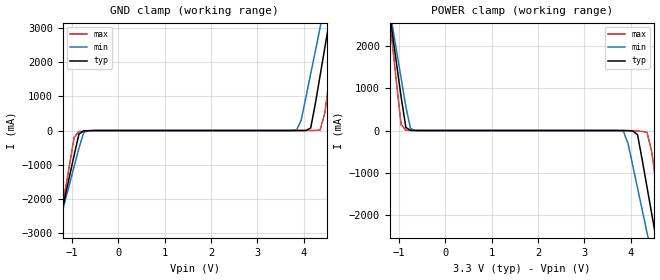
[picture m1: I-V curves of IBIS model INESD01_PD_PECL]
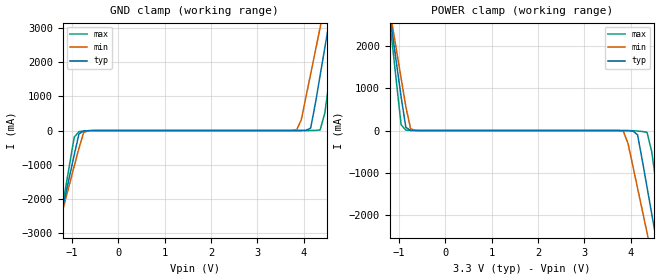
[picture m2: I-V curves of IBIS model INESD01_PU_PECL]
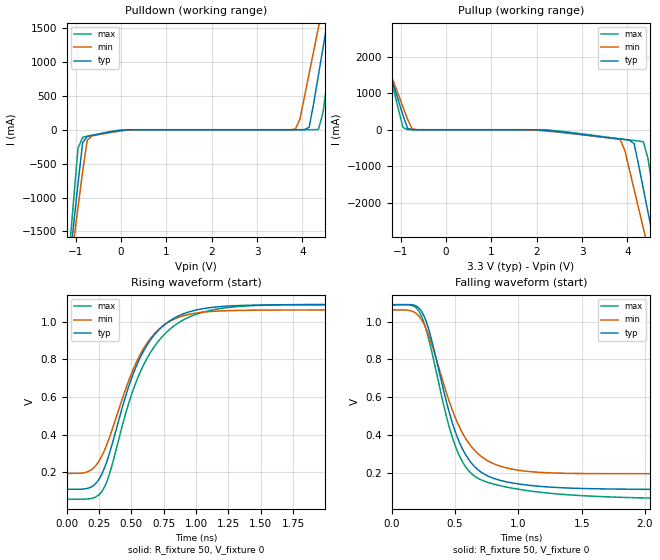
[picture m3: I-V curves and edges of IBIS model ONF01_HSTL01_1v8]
|   This file is an IBIS representation of the   |
|   Integrated Device Technology , Inc.   |
|   ICS8725-21   |
|   DIFFERENTIAL-TO-HSTL ZERO DELAY CLOCK GENERATOR   |
[IBIS Ver]   4.1
[File name]   8725_21_3v3.ibs
[File Rev]   2.0
[Date]   2 Sep 2009 | Last modified
|   2 Jul 2002 | Generated
[Source]   Originated at Integrated Device Technology, Inc.
[Disclaimer]
IDT hereby grants the user of this IBIS model a non-exclusive,
nontransferable license to use this IBIS model under the following terms.
Before using this IBIS model, the user should read this license.
If the user does not accept these terms,  the IBIS model should be
returned to IDT within 30 days.
   The user is granted this license only to use the IBIS model and
is not granted rights to sell, load, rent, lease or license the IBIS
model in whole or in part, or in modified form to anyone other than
user. User may modify the IBIS model to suit its specific
applications but rights to derivative works and such modifications
shall belong to IDT.
   This IBIS model is provided on an "AS IS" basis and IDT makes
absolutely no warranty with respect to the information contained
herein. IDT DISCLAIMS AND CUSTOMER WAIVES ALL WARRANTIES, EXPRESS
OR IMPLIED, INCLUDING WARRANTIES OF MERCHANTABILITY OR FITNESS FOR
A PARTICULAR PURPOSE. The entire risk as to quality and performance
is with the Customer. ACCORDINGLY, IN NO EVENT SHALL THE COMPANY BE
LIABLE FOR ANY DAMAGES, WHETHER IN CONTRACT OR TORT,INCLUDING ANY
LOST PROFITS OR OTHER INCIDENTAL, CONSEQUENTIAL, EXEMPLARY, OR
PUNITIVE DAMAGES ARISING OUT OF THE USE OR APPLICATION OF THE IBIS
model provided in this package. Further, IDT reserves the right to
make changes without notice to any product herein to improve
reliability, function, or design. IDT does not convey any license
under patent rights or any other intellectual property rights,
including those of third parties.
   IDT is not obligated to provide maintenance or support
for the licensed IBIS model.
[Copyright]   Copyright 2002 by Integrated Device Technology , Inc.
[Component]   8725M_21
[Manufacturer] Integrated Device Technology, Inc.
[Package]
|SOIC 20 Lead
|   typ   min   max
R_pkg   57.15m   45.4m   68.9m
L_pkg   4.051n   2.187n   5.914n
C_pkg   0.796p   0.419p   1.173p
[Pin]  signal_name   model_name   R_pin   L_pin   C_pin
1   CLK   INESD01_PD_PECL   68.90m   5.914n   1.173p
2   nCLK   INESD01_PU_PECL   63.02m   4.983n   0.985p
3   MR   INESD01_PD_PECL   57.15m   4.051n   0.796p
4   VDD   POWER   51.25m   3.119n   0.608p
5   nFB_IN   INESD01_PU_PECL   45.40m   2.187n   0.419p
6   FB_IN   INESD01_PD_PECL   45.40m   2.187n   0.419p
7   SEL2   INESD01_PD_PECL   51.25m   3.119n   0.608p
8   GND   GND   57.15m   4.051n   0.796p
9   nQFB   ONF01_HSTL01_1v8   63.02m   4.983n   0.985p
10   QFB   ONF01_HSTL01_1v8   68.90m   5.914n   1.173p
11   nQ   ONF01_HSTL01_1v8   68.90m   5.914n   1.173p
12   Q   ONF01_HSTL01_1v8   63.02m   4.983n   0.985p
13   VDDO   POWER   57.15m   4.051n   0.796p
14   SEL3   INESD01_PD_PECL   51.25m   3.119n   0.608p
15   VDDA   POWER   45.40m   2.187n   0.419p
16   PLL_SEL   INESD01_PU_PECL   45.40m   2.187n   0.419p
17   VDD   POWER   51.25m   3.119n   0.608p
18   SEL0   INESD01_PD_PECL   57.15m   4.051n   0.796p
19   SEL1   INESD01_PD_PECL   63.02m   4.983n   0.985p
20   NC   NC   68.90m   5.914n   1.173p
[Diff Pin]  inv_pin  vdiff tdelay_typ tdelay_min  tdelay_max
|Output
10   9   NA   0   0   0
12   11   NA   0   0   0
|Input
1   2   0.15   0   0   0
6   5   0.15   0   0   0
| Models and submodels in the file (3): INESD01_PD_PECL (Input), INESD01_PU_PECL (Input), ONF01_HSTL01_1v8 (Output)
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[Model]   INESD01_PD_PECL
Model_type  Input
Polarity   Non-Inverting
Vinl = 0.8V
Vinh = 2.0V
|   typ   min   max
C_comp   2pF   1.5pF   2.5pF
|   typ   min   max
[Voltage range]  3.3V   3.15V   3.45V
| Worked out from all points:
|   GND clamp passes 1 mA (typ) near -0.55 V on its own axis
|   POWER clamp passes 1 mA (typ) near -0.66 V on its own axis
[GND_clamp]
|Voltage   I(typ)   I(min)   I(max)
-2.586V   -10.86A    -9.487A    -13.15A
-1.361V   -3.24A     -3.145A    -3.432A
-1.259V   -2.606A    -2.617A    -2.622A
-952.6mV  -705.3mA   -1.038A    -192.4mA
-850.5mV  -99.9mA    -513.5mA   -31.23mA
-646.4mV  -3.788mA   -3.549mA   -8.297mA
3.844V    129.1uA    13.13mA    71.12uA
4.151V    73.33mA    1.652A     864.7uA
4.355V    1.607A     3.003A     15.44mA
4.559V    3.233A     4.356A     1.553A
4.763V    4.861A     5.711A     3.635A
5.375V    9.757A     9.783A     9.893A
[POWER_clamp]
|Voltage   I(typ)   I(min)   I(max)
-2.177V   10.57A     9.364A     12.62A
-1.157V   2.42A      2.586A     2.194A
-952.6mV  795.8mA    1.237A     137.8mA
-850.5mV  73.33mA    563.2mA    8.145mA
-646.4mV  535.8uA    2.004mA    431.2uA
3.844V    -826.3uA   -18.14mA   -47.07uA
4.151V    -99.9mA    -1.362A    -11.82mA
4.355V    -1.338A    -2.415A    -41.71mA
4.559V    -2.606A    -3.47A     -1.312A
4.661V    -3.24A     -3.998A    -2.123A
4.763V    -3.875A    -4.526A    -2.933A
5.579V    -8.954A    -8.756A    -9.414A
[Model]   INESD01_PU_PECL
Model_type  Input
Polarity   Non-Inverting
Vinl = 0.8V
Vinh = 2.0V
|   typ   min   max
C_comp   2pF   1.5pF   2.5pF
|   typ   min   max
[Voltage range]  3.3V   3.15V   3.45V
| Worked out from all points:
|   GND clamp passes 1 mA (typ) near -0.55 V on its own axis
|   POWER clamp passes 1 mA (typ) near -0.67 V on its own axis
[GND_clamp]
|Voltage   I(typ)   I(min)   I(max)
-3.3V     -15.3A     -13.19A    -18.82A
-1.361V   -3.24A     -3.145A    -3.432A
-1.259V   -2.606A    -2.617A    -2.622A
-952.6mV  -705.4mA   -1.038A    -192.5mA
-850.5mV  -99.96mA   -513.6mA   -31.29mA
-646.4mV  -3.852mA   -3.611mA   -8.361mA
3.844V    64.83uA    13.07mA    7.183uA
4.151V    73.26mA    1.652A     800.8uA
4.355V    1.607A     3.003A     15.37mA
4.559V    3.233A     4.356A     1.553A
4.763V    4.861A     5.711A     3.635A
6.6V      19.56A     17.94A     22.42A
[POWER_clamp]
|Voltage   I(typ)   I(min)   I(max)
-3.3V     19.56A     16.84A     24.11A
-1.259V   3.233A     3.262A     3.235A
-1.157V   2.419A     2.586A     2.194A
-952.6mV  795.8mA    1.236A     137.7mA
-850.5mV  73.26mA    563.1mA    8.081mA
-646.4mV  471.5uA    1.942mA    367.2uA
3.844V    -890.5uA   -18.21mA   -111uA
4.151V    -99.96mA   -1.362A    -11.88mA
4.355V    -1.338A    -2.415A    -41.77mA
4.559V    -2.606A    -3.47A     -1.313A
4.763V    -3.875A    -4.526A    -2.933A
6.6V      -15.3A     -14.05A    -17.51A
[Model]   ONF01_HSTL01_1v8
|3.3V core, 1.8V output supply
Model_type  Output
Polarity   Non-Inverting
Vmeas = .6
Rref = 50
Cref = 0
Vref = 0
|Variable  typ   min   max
C_comp   2p   1.5p   2.5p
[Voltage Range]   3.3   3.135   3.465
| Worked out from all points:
|   slope of the pulldown table from 0 to 0.495 V, typ, clamps not added: 54.9 ohm
|   rising waveform, R_fixture 50, V_fixture 0: 20-80 % time 306ps typ, 302ps min, 333ps max; typ from 0.111 V to 1.09 V
|   falling waveform, R_fixture 50, V_fixture 0: 20-80 % time 255ps typ, 284ps min, 252ps max; typ from 1.09 V to 0.111 V
| Open source, no load
|  Voltage   I(typ)   I(min)   I(max)
[Pulldown]
-3.3V     -15.42A    -13.35A    -18.91A
-1.157V   -2.072A    -2.21A     -1.894A
-1.055V   -1.436A    -1.68A     -1.084A
-952.6mV  -800.4mA   -1.149A    -274.1mA
-850.5mV  -191.4mA   -618.4mA   -111.9mA
-544.3mV  -70.23mA   -78.22mA   -68.72mA
3.844V    27.09uA    7.698mA    3.013nA
4.151V    36.63mA    830.7mA    49.54uA
4.355V    803.8mA    1.508A     4.53mA
4.559V    1.617A     2.187A     770.5mA
4.763V    2.432A     2.867A     1.809A
6.6V      9.786A     9.002A     11.19A
[Pullup]
-3.3V     9.786A     8.45A      12.03A
-1.565V   2.839A     2.657A     3.17A
-1.463V   2.432A     2.317A     2.65A
-952.6mV  398mA      622.1mA    64.71mA
-850.5mV  36.63mA    284.2mA    1.532mA
-646.4mV  229.4uA    1.613mA    19.07uA
3.844V    -256mA     -270.5mA   -249.6mA
4.151V    -379.9mA   -1.636A    -294.5mA
4.355V    -1.626A    -2.699A    -329.8mA
4.559V    -2.898A    -3.761A    -1.602A
4.763V    -4.17A     -4.823A    -3.222A
6.6V      -15.62A    -14.38A    -17.8A
[Ramp]
|   typ   min   max
dV/dt_r   0.782/0.488n   0.693/0.472n   0.826/0.535n
dV/dt_f   0.783/0.418n   0.693/0.453n   0.822/0.447n
R_load =   50.0000
[Rising Waveform]
R_fixture = 50
V_fixture = 0
C_fixture = 0.0p
| Time   typ   min   max
0s        110.9mV    195.1mV    57.72mV
173.6ps   118.9mV    207.8mV    60.43mV
275.9ps   199mV      294.5mV    104.4mV
334.8ps   312.4mV    395.2mV    202.7mV
480.5ps   659.8mV    690.1mV    570.6mV
579.7ps   826mV      840.3mV    750.2mV
728.5ps   967.2mV    969.3mV    912.9mV
917.6ps   1.045V     1.034V     1.015V
1.423ns   1.087V     1.06V      1.084V
2.998ns   1.089V     1.062V     1.089V
[Falling Waveform]
R_fixture = 50
V_fixture = 0
C_fixture = 0.0p
| Time   typ   min   max
0s        1.089V     1.062V     1.088V
170.5ps   1.087V     1.052V     1.083V
244.9ps   1.042V     999.2mV    1.011V
303.8ps   931.1mV    904.4mV    875.3mV
421.6ps   601.8mV    644.6mV    525.1mV
492.9ps   434.4mV    506.4mV    359mV
582.8ps   296.3mV    382.4mV    232.4mV
691.3ps   210.9mV    295.1mV    167.5mV
1.163ns   128.8mV    202.7mV    97.96mV
2.998ns   111.1mV    195.1mV    59.79mV
